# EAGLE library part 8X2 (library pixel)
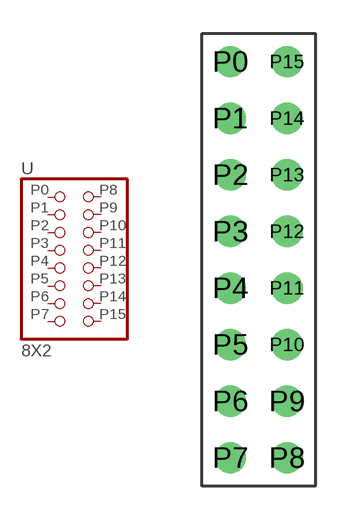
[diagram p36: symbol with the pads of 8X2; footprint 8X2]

Designator prefix -

## 8X2  [8X2]
P0  P0  pas
P1  P1  pas
P2  P2  pas
P3  P3  pas
P4  P4  pas
P5  P5  pas
P6  P6  pas
P7  P7  pas
P8  P8  pas
P9  P9  pas
P10  P10  pas
P11  P11  pas
P12  P12  pas
P13  P13  pas
P14  P14  pas
P15  P15  pas

## Footprint 8X2 (pad centres in mm)
drill 0.9 pad 1.27: P0 -1.27,8.89; P1 -1.27,6.35; P2 -1.27,3.81; P3 -1.27,1.27; P4 -1.27,-1.27; P5 -1.27,-3.81; P6 -1.27,-6.35; P7 -1.27,-8.89; P8 1.27,-8.89; P9 1.27,-6.35; P10 1.27,-3.81; P11 1.27,-1.27; P12 1.27,1.27; P13 1.27,3.81; P14 1.27,6.35; P15 1.27,8.89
